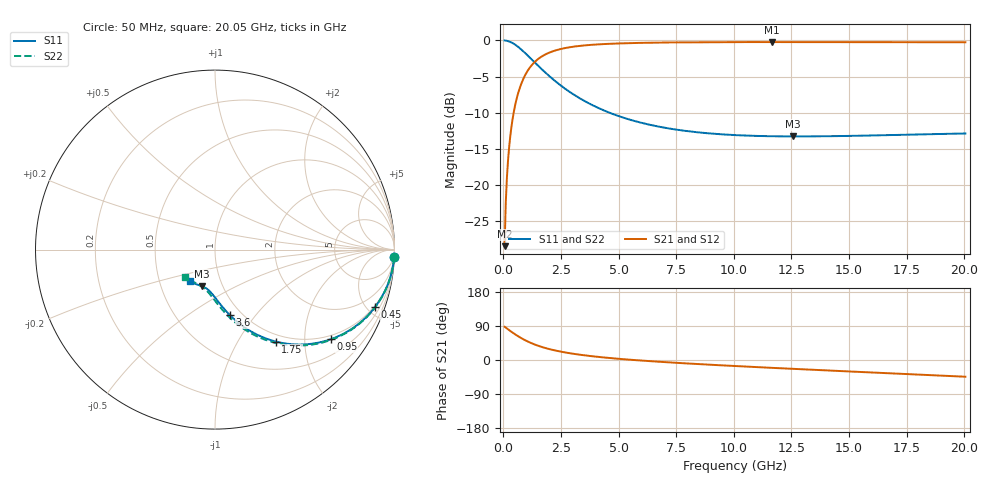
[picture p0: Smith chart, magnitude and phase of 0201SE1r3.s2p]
! AVX Thin Film Operation		Date: August 2001
! Description: Accu-P® Series, Thin Film, SMD, RF Capacitor
! Part Number: 02013J1R3ABW
! 50 MHz  -  20.05 GHz
! Serial Measurements
# mhz S db R 50
!	S11		S21		S12		S22
!	dB	Phase	dB	Phase	dB	Phase	dB	Phase
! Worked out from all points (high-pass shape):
!   401 points, 50 MHz to 20.05 GHz, reference 50 ohm
!   highest |S21| = -0.23 dB at 11.65 GHz (marker M1); lowest = -28.5 dB at 50 MHz (marker M2)
!   |S21| within 3 dB of the highest: 1.284 GHz to end of sweep
!   lowest |S11| = -13.3 dB at 12.55 GHz (marker M3), VSWR 1.55, Z = 40 - j17.1 ohm
!   |S11| at or under -10 dB: 4.591 GHz to end of sweep
!   |S22| runs from -13.3 to 0.0 dB; largest |S21 - S12| = 0
!   S11 on the Smith chart (normalised r, x): 50 MHz: 1, -50; 450 MHz: 0.89, -5.58; 950 MHz: 0.89, -2.66; 1.75 GHz: 0.89, -1.46; 3.6 GHz: 0.88, -0.75; 20.05 GHz: 0.71, -0.26
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50  -0.01 -2.3  -28.50 87.7  -28.50 87.7  -0.01 -2.3
100  -0.03 -4.6  -22.50 85.4  -22.50 85.4  -0.03 -4.6
200  -0.10 -9.1  -16.56 80.9  -16.56 80.9  -0.10 -9.2
250  -0.15 -11.3  -14.67 78.6  -14.67 78.6  -0.15 -11.4
350  -0.29 -15.6  -11.89 74.2  -11.89 74.2  -0.29 -15.8
450  -0.47 -19.8  -9.89 70.0  -9.89 70.0  -0.47 -20.1
650  -0.93 -27.7  -7.17 62.1  -7.17 62.1  -0.93 -28.0
950  -1.77 -37.8  -4.75 51.9  -4.75 51.9  -1.77 -38.3
1300  -2.87 -47.3  -3.17 42.2  -3.17 42.2  -2.87 -48.0
1750  -4.25 -56.6  -2.06 32.8  -2.06 32.8  -4.25 -57.6
2100  -5.25 -62.2  -1.55 27.1  -1.55 27.1  -5.25 -63.3
2450  -6.15 -66.7  -1.22 22.5  -1.22 22.5  -6.15 -68.0
3400  -8.18 -75.7  -0.73 13.2  -0.73 13.2  -8.18 -77.5
3600  -8.54 -77.2  -0.67 11.7  -0.67 11.7  -8.54 -79.1
5050  -10.54 -85.6  -0.41 2.9  -0.41 2.9  -10.54 -88.2
6750  -11.95 -92.6  -0.30 -4.6  -0.30 -4.6  -11.96 -96.0
10050  -13.12 -102.9  -0.23 -15.9  -0.23 -15.9  -13.14 -107.9
11650  -13.28 -107.3  -0.23 -20.7  -0.23 -20.7  -13.31 -113.0
12550  -13.30 -109.7  -0.23 -23.3  -0.23 -23.3  -13.34 -115.8
13400  -13.29 -112.0  -0.23 -25.7  -0.23 -25.7  -13.33 -118.4
16750  -13.12 -120.5  -0.24 -35.0  -0.24 -35.0  -13.17 -128.4
20050  -12.89 -128.8  -0.26 -44.1  -0.26 -44.1  -12.96 -138.1
